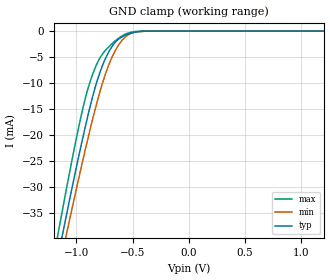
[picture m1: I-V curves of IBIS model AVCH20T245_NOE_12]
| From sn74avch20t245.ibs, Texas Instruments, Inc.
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[Model]   AVCH20T245_NOE_12
Model_type  Input
Vinl=0.385
Vinh=0.845
| variable   typ   min   max
C_comp   2.92pF   2.54pF   3.33pF
[Temperature Range]   40   100   -40
| Ambient temperature   25   85   -40
[Voltage range]   1.2   1.1   1.3
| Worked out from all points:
|   GND clamp passes 1 mA (typ) near -0.58 V on its own axis
[GND Clamp]
| AVCH20T245_NOE_12
|   Voltage   I(typ)   I(min)   I(max)
-4.6V     -459.2mA   -437.9mA   -484.2mA
-1.165V   -43.78mA   -47mA      -39.35mA
-1.115V   -38.35mA   -41.89mA   -33.51mA
-1.09V    -35.67mA   -39.36mA   -30.63mA
-1.065V   -33.02mA   -36.85mA   -27.8mA
-945mV    -20.79mA   -25.16mA   -15.18mA
-840mV    -11.44mA   -15.71mA   -7.485mA
-710mV    -3.942mA   -6.433mA   -2.997mA
-630mV    -1.665mA   -2.889mA   -1.475mA
-555mV    -700.6uA   -964.8uA   -509.7uA
-385mV    -23.61uA   -32.06uA   -5.101uA
1.2V      106.8pA    765.6pA    17.5pA
